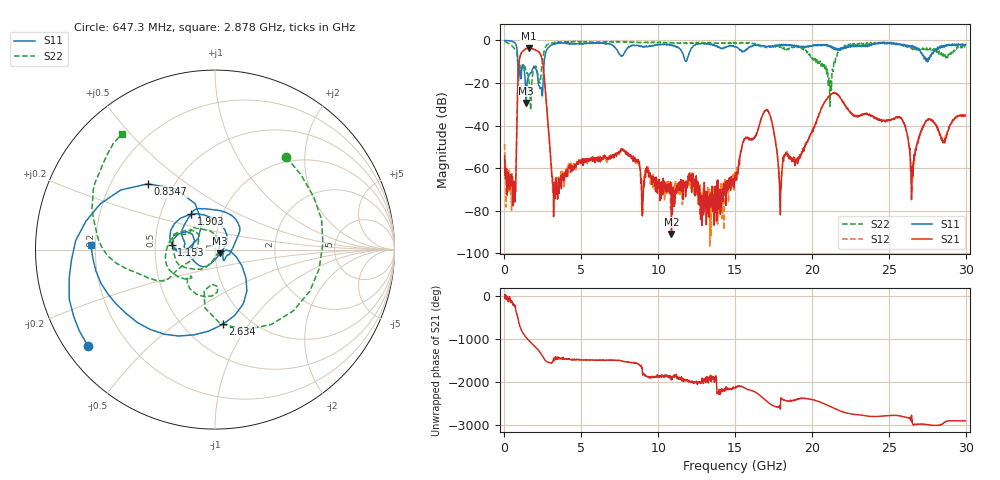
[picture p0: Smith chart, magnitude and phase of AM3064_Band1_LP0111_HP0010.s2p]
# Hz S DB R 50.0
!freq dBS11 angS11 dBS21 angS21 dBS12 angS12 dBS22 angS22
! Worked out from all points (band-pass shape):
!   1600 points, 10 MHz to 29.98 GHz, reference 50 ohm
!   highest |S21| = -3.65 dB at 1.584 GHz (marker M1); lowest = -91.0 dB at 10.86 GHz (marker M2)
!   |S21| within 3 dB of the highest: 1.05 GHz to 2.346 GHz (1.295 GHz wide, 76.3 % of centre)
!   lowest |S11| = -29.4 dB at 1.416 GHz (marker M3), VSWR 1.07, Z = 52.7 - j2.2 ohm
!   |S11| at or under -10 dB: 865.8 MHz to 2.588 GHz (1.722 GHz wide, 99.7 % of centre); 27.52381 GHz to 27.53639 GHz (12.58 MHz wide, 0.0457 % of centre)
!   |S22| runs from -32.8 to -0.3 dB; largest |S21 - S12| = 0.0089
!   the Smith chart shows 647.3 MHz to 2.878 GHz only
!   S11 on the Smith chart (normalised r, x): 647.3 MHz: 0.07, -0.33; 834.7 MHz: 0.36, +0.36; 1.153 GHz: 0.61, +0.03; 1.903 GHz: 0.71, +0.30; 2.634 GHz: 0.76, -0.77; 2.878 GHz: 0.18, +0.02
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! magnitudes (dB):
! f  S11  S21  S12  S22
! 10 MHz  0.0  -54.4  -48.7  -0.3
! 647.3 MHz  -1.0  -68.9  -69.7  -3.7
! 834.7 MHz  -5.6  -30.2  -30.2  -7.7
! 1.153 GHz  -12.3  -5.4  -5.3  -12.0
! 1.416 GHz  -29.4  -3.9  -3.8  -15.4
! 1.584 GHz  -16.4  -3.6  -3.7  -18.6
! 1.903 GHz  -12.5  -4.2  -4.1  -13.2
! 2.634 GHz  -7.6  -21.1  -21.0  -3.7
! 2.878 GHz  -3.2  -43.4  -43.3  -1.6
! 3.309 GHz  -1.6  -74.4  -71.7  -1.2
! 5.015 GHz  -1.4  -56.0  -57.4  -0.7
! 10 GHz  -2.0  -66.3  -65.7  -1.0
! 10.86 GHz  -2.3  -91.0  -66.9  -1.1
! 15 GHz  -2.9  -65.0  -64.0  -1.5
! 16.99 GHz  -2.9  -32.8  -32.7  -3.1
! 17.93 GHz  -2.0  -70.4  -78.1  -2.6
! 19.99 GHz  -2.8  -43.3  -42.8  -8.1
! 21.43 GHz  -4.2  -24.8  -24.5  -10.1
! 25 GHz  -1.0  -37.4  -37.5  -1.2
! 26.53 GHz  -2.4  -59.5  -57.7  -4.2
! 27.47 GHz  -8.5  -37.6  -37.3  -3.6
! 29.98 GHz  -1.9  -35.5  -35.2  -2.8
